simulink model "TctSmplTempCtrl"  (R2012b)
settings: Solver=ode3  SolverMode=SingleTasking  StartTime=0.0  StopTime=10  FixedStep=0.005  RelTol=1e-3
PostLoadFcn:
  | load('TctSmplTempCtrlParameters.mat');
  | load('TctSmplTempCtrlBusObjects.mat');
undefined symbols (not defined in the file): Kp, Tn, y_max, y_min
libraries: simulink x1

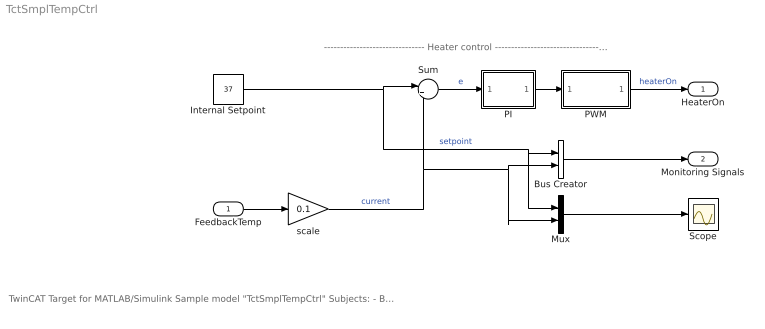
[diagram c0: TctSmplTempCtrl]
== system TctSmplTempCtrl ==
  note: ------------------------------- Heater control ------------------------------------------------------------------------------------------
  note: TwinCAT Target for MATLAB/Simulink Sample model "TctSmplTempCtrl" Subjects: - Basics - BusObjects - Testpoints - External Mode
  FeedbackTemp : Inport  OutDataTypeStr=int16
  Bus Creator : BusCreator  Inputs=2  OutDataTypeStr=Bus: MonitoringSignalsType
  Internal Setpoint : Constant  Value=37
  Mux : Mux  Inputs=2
  PI : Subsystem
  PWM : Subsystem
  Scope : Scope
  Sum : Sum  Inputs=|+-
  scale : Gain  Gain=0.1  ParamDataTypeStr=double
  HeaterOn : Outport  OutDataTypeStr=boolean
  Monitoring Signals : Outport  Port=2  OutDataTypeStr=Bus: MonitoringSignalsType
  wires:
  Sum/1 -> PI/1(e)  "e"
  PI/1(y) -> PWM/1(Value)
  FeedbackTemp/1 -> scale/1
  scale/1 -> Sum/2, Mux/2, Bus Creator/2  "current"
  PWM/1(PWM) -> HeaterOn/1  "heaterOn"
  Internal Setpoint/1 -> Sum/1, Mux/1, Bus Creator/1  "setpoint"
  Mux/1 -> Scope/1
  Bus Creator/1 -> Monitoring Signals/1

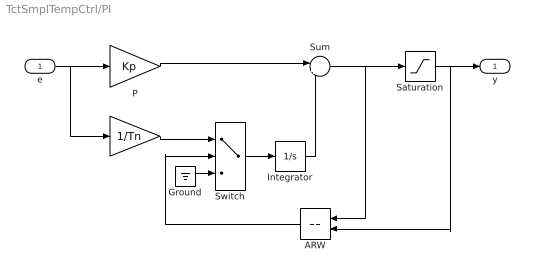
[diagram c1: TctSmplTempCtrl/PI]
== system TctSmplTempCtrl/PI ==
  e : Inport
  ARW : RelationalOperator  Operator===  OutDataTypeStr=boolean
  Ground : Ground
  I : Gain  Gain=1/Tn
  Integrator : Integrator
  P : Gain  Gain=Kp
  Saturation : Saturate  UpperLimit=y_max  LowerLimit=y_min
  Sum : Sum  Inputs=|++
  Switch : Switch  Criteria=u2 > Threshold
  y : Outport
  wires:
  e/1 -> P/1, I/1
  Integrator/1 -> Sum/2
  P/1 -> Sum/1
  Sum/1 -> Saturation/1, ARW/1
  Saturation/1 -> y/1, ARW/2
  Switch/1 -> Integrator/1
  ARW/1 -> Switch/2
  I/1 -> Switch/1
  Ground/1 -> Switch/3

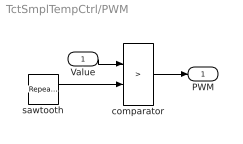
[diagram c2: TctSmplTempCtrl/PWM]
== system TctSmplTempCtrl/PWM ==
  Value : Inport  OutDataTypeStr=double
  comparator : RelationalOperator  Operator=>  OutDataTypeStr=boolean
  sawtooth : simulink/Sources/Repeating Sequence  rep_seq_t=[0 .1]  rep_seq_y=[0 60]
  PWM : Outport  OutDataTypeStr=boolean
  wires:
  Value/1 -> comparator/1
  sawtooth/1 -> comparator/2
  comparator/1 -> PWM/1
